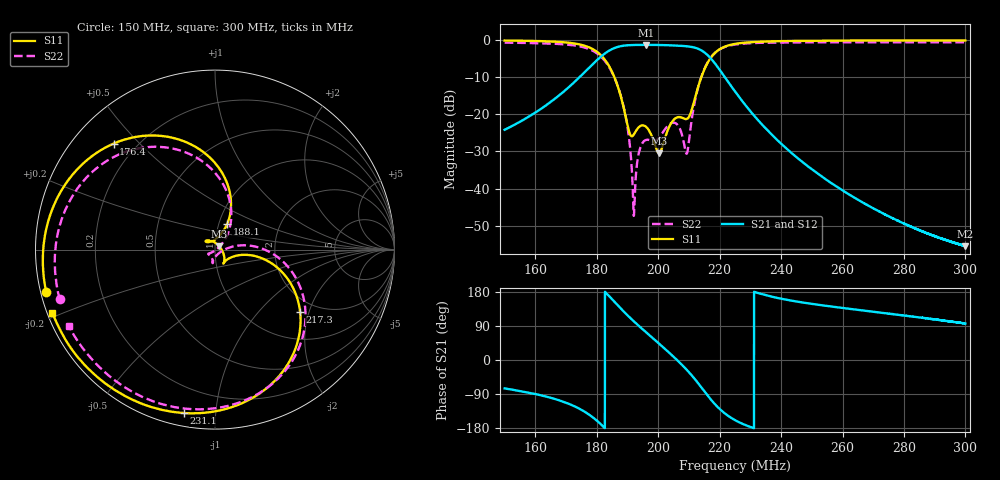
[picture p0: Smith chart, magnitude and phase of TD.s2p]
#  HZ  S  DB  R  50.00
! Rohde & Schwarz Vector Network Analyzer
! Rohde-Schwarz,ZNL6-2Port,1323001206101378,1.50.1.34-21.10.1.104
! Created: UTC 4/19/2023, 7:42:05 AM
! freq[Hz]  db:S11  ang:S11  db:S21  ang:S21  db:S12  ang:S12  db:S22  ang:S22
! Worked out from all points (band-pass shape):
!   5001 points, 150 MHz to 300 MHz, reference 50 ohm
!   highest |S21| = -1.43 dB at 196 MHz (marker M1); lowest = -55.5 dB at 300 MHz (marker M2)
!   |S21| within 3 dB of the highest: 181.6 MHz to 216.4 MHz (34.82 MHz wide, 17.5 % of centre)
!   lowest |S11| = -30.5 dB at 200.3 MHz (marker M3), VSWR 1.06, Z = 52.2 + j2.09 ohm
!   |S11| at or under -10 dB: 185.7 MHz to 214.1 MHz (28.38 MHz wide, 14.2 % of centre)
!   |S22| runs from -47.3 to -0.7 dB; largest |S21 - S12| = 0.01
!   S11 on the Smith chart (normalised r, x): 150 MHz: 0.02, -0.12; 176.4 MHz: 0.12, +0.42; 188.1 MHz: 1.10, +0.32; 217.3 MHz: 1.65, -1.75; 231.1 MHz: 0.06, -0.83; 300 MHz: 0.01, -0.19
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1.5e8  -0.27 -166.0  -24.21 -75.0  -24.19 -76.0  -0.84 -162.2
1.6584e8  -0.54 168.6  -16.22 -101.7  -16.22 -102.7  -1.12 173.4
1.7502e8  -1.42 140.1  -9.58 -131.6  -9.57 -132.5  -1.93 145.6
1.7643e8  -1.75 133.7  -8.44 -138.4  -8.42 -139.3  -2.24 139.2
1.803e8  -3.43 111.7  -5.34 -161.9  -5.33 -162.7  -3.84 117.2
1.8372e8  -6.73 87.8  -3.13 171.2  -3.13 170.5  -7.00 92.2
1.8807e8  -15.98 64.6  -1.73 133.7  -1.74 133.1  -15.81 58.1
1.9023e8  -23.75 80.9  -1.52 116.1  -1.53 115.5  -24.71 41.2
1.9206e8  -25.48 126.9  -1.45 102.0  -1.47 101.5  -47.34 -53.1
1.9386e8  -23.39 139.5  -1.43 88.8  -1.44 88.3  -29.87 -143.7
1.9599e8  -23.39 130.6  -1.43 73.6  -1.44 73.1  -26.94 -148.0
2.0001e8  -30.37 53.4  -1.45 45.1  -1.46 44.5  -26.60 -116.7
2.0028e8  -30.50 42.2  -1.45 43.2  -1.47 42.6  -26.35 -113.9
2.0547e8  -21.22 -54.6  -1.60 5.0  -1.61 4.4  -22.38 -100.3
2.0934e8  -21.31 -43.9  -1.80 -26.3  -1.82 -27.0  -30.58 -43.0
2.1297e8  -12.80 -9.2  -2.46 -60.9  -2.49 -61.7  -12.92 4.2
2.1735e8  -4.62 -36.2  -5.28 -106.3  -5.32 -107.2  -4.57 -32.0
2.25e8  -1.16 -81.6  -13.93 -158.6  -13.97 -160.0  -1.34 -79.2
2.3109e8  -0.66 -100.8  -20.31 -179.7  -20.34 178.7  -0.93 -98.2
2.5002e8  -0.32 -129.5  -34.83 148.1  -34.87 146.4  -0.74 -125.9
2.7501e8  -0.24 -147.2  -47.45 122.4  -47.51 120.2  -0.73 -142.8
3e8  -0.24 -158.8  -55.47 96.2  -55.46 94.1  -0.74 -152.5
